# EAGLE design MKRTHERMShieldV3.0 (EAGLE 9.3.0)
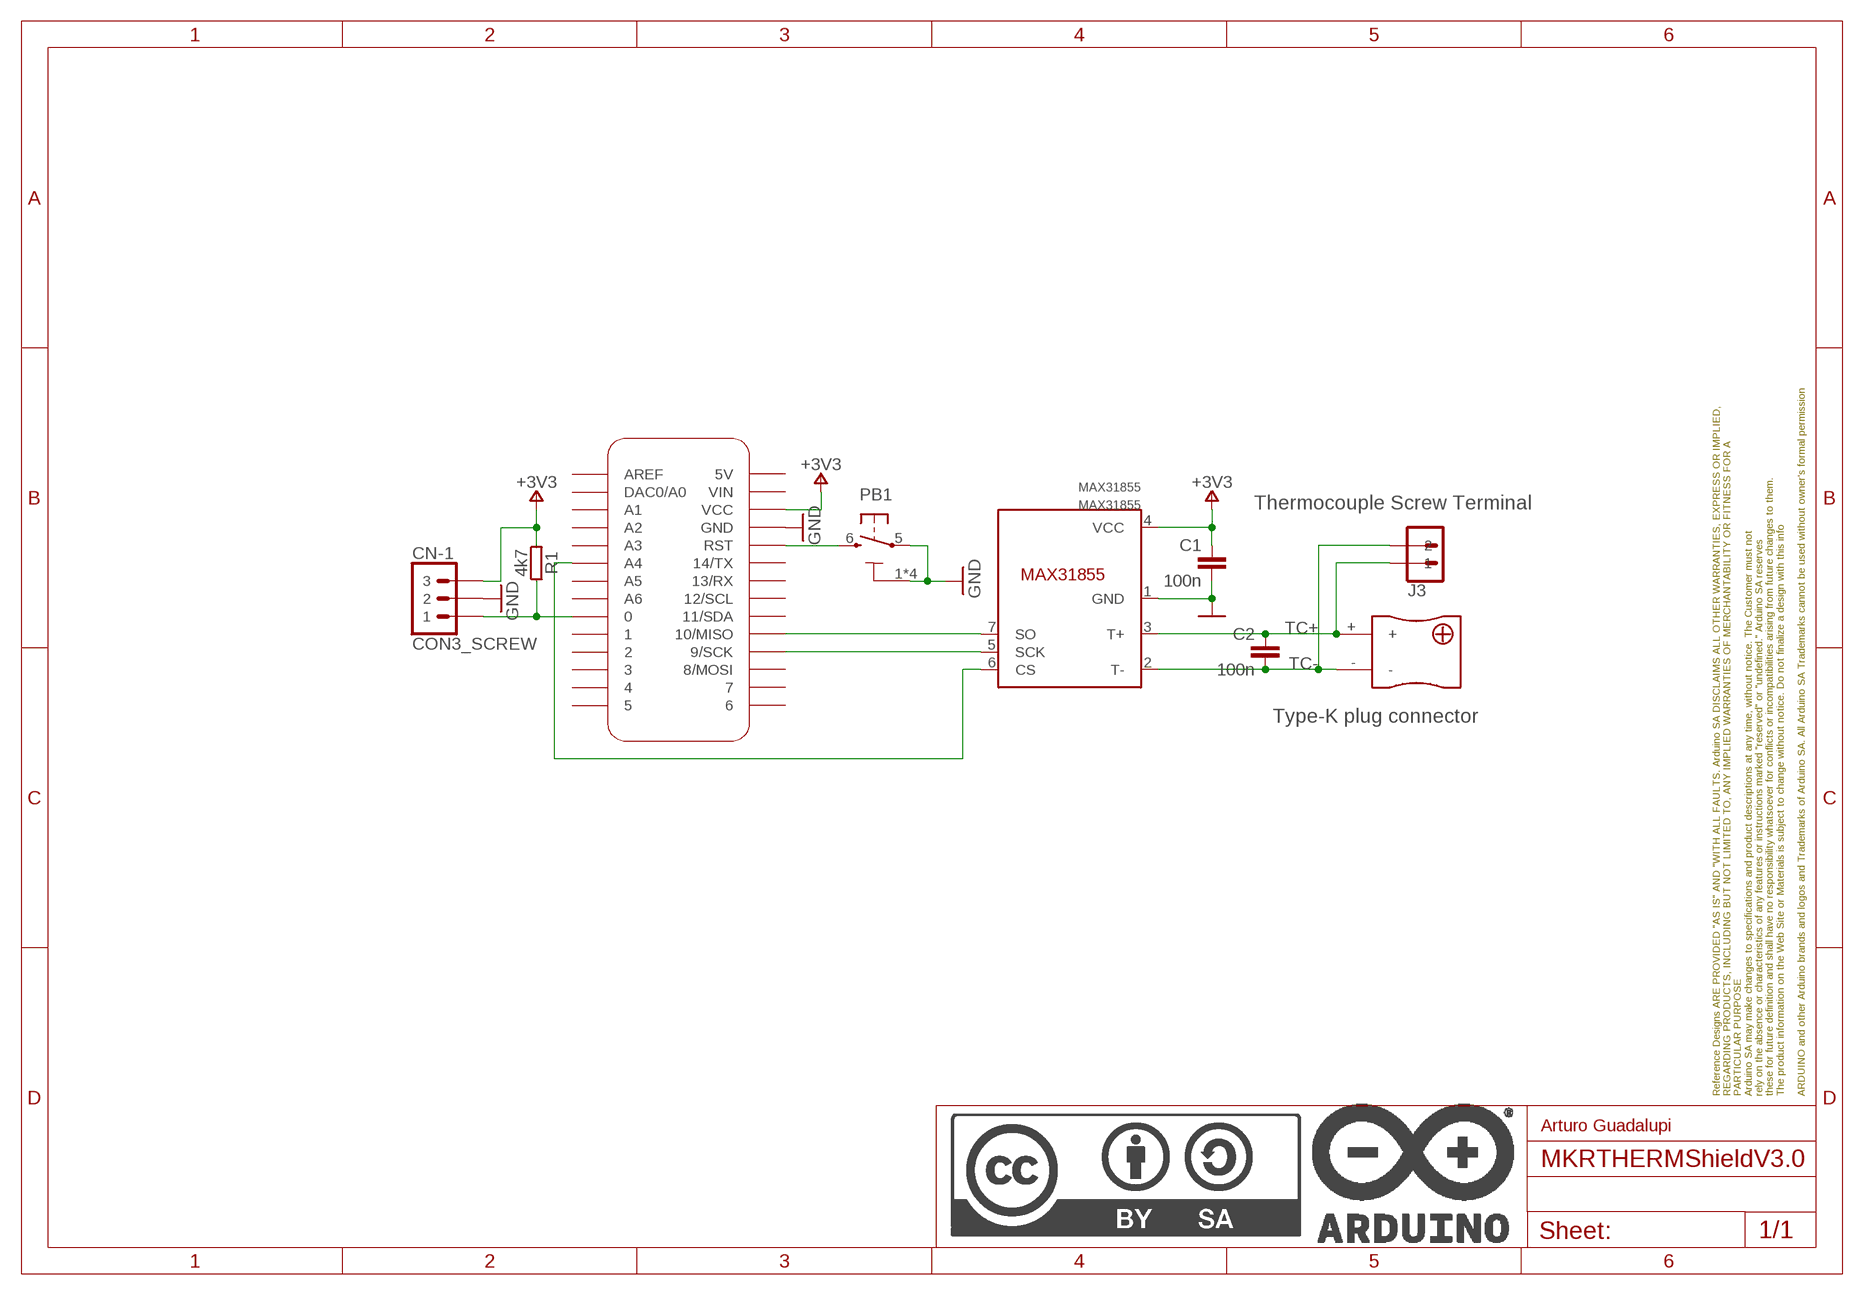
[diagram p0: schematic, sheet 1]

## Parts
C1  100n  C-100NF-0402  [0402-1005X55N]
C2  100n  C-100NF-0402  [0402-1005X55N]
CN-1  CON3_SCREW  SCREW_1X03_254MM  [1X03_2.54_SCREWTERM_FT]
FRAME1  DNP  A4L-LOC  [FRAME]
J3  SCREW2X8.25_  [1X02_8.25_BARRIER-TERMINAL]
MAX31855  MAX31855  [SOIC8]
MKR1  -  MKRBOARD-SHORTTEXT  [MKRBOARD-DIM-SHORTTEXT]
PB1  PTS820  TACTILE1PTS820-NH  [C&K_PTS820_NO_HOLES]
R1  4k7  R-4K7-0402  [0402-1005X55N]
U$1  THERMO_K-PLUG-PCB  [THERMO_K-PLUG-PCB]

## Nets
+3V3: C1.1 CN-1.P$3 MAX31855.4(VCC) MKR1.VCC R1.2
DS18X_DATA: CN-1.P$1 MKR1.0 R1.1
GND: C1.2 CN-1.P$2 MAX31855.1(GND) MKR1.GND PB1.1 PB1.2 PB1.3 PB1.4 PB1.5
MISO: MAX31855.7(SO) MKR1.10(10/MISO)
RESET: MKR1.RST PB1.6
SCK: MAX31855.5(SCK) MKR1.9(9/SCK)
TC+: C2.1 J3.P$1 MAX31855.3(T+) U$1.+
TC-: C2.2 J3.P$2 MAX31855.2(T-) U$1.-
THERMO_CS: MAX31855.6(CS) MKR1.A4
Unconnected: MKR1.1 MKR1.2 MKR1.3 MKR1.4 MKR1.5 MKR1.5V MKR1.6 MKR1.7 MKR1.8(8/MOSI) MKR1.11(11/SDA) MKR1.12(12/SCL) MKR1.13(13/RX) MKR1.14(14/TX) MKR1.A0(DAC0/A0) MKR1.A1 MKR1.A2 MKR1.A3 MKR1.A5 MKR1.A6 MKR1.AREF MKR1.VIN

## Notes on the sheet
- Thermocouple Screw Terminal
- Type-K plug connector
- Arturo Guadalupi

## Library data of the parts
C1 C2 = Arduino-rcl:C: SMD Capacitor; CODE-ARDUINO: 0132; DATASHEET: http://www.tdk.com/pdf/TDKMLCCCapRange.pdf; DISTRIBUTOR-LINK: http://www.digikey.com/product-detail/en/tdk-corporation/C1005X5R1H104K050BB/445-5942-1-ND/2443982; DISTRIBUTOR-PN: 445-5942-1-ND; MANUFACTURER: TDK; MANUFACTURER-PN: C1005X5R1H104K050BB; NOTE: -
CN-1 = Arduino-connectors:SCREW_1X03_254MM; CODE-ARDUINO: -; DATASHEET: http://www.te.com/commerce/DocumentDelivery/DDEController?Action=srchrtrv&DocNm=282834&DocType=Customer+Drawing&DocLang=English; DISTRIBUTOR-LINK: https://www.digikey.com/product-detail/en/te-connectivity-amp-connectors/282834-3/A98334-ND/1153264; DISTRIBUTOR-PN: A98334-ND; MANUFACTURER: TE Connectivity; MANUFACTURER-PN: 282834-3
FRAME1 = Arduino-utility:A4L-LOC; CODE-ARDUINO: DNP; DATASHEET: DNP; DISTRIBUTOR-LINK: DNP; DISTRIBUTOR-PN: DNP; MANUFACTURER: DNP; MANUFACTURER-PN: DNP; NOTE: DNP
J3 = Arduino-connectors:SCREW2X8.25: AdamTech Terminal Barrier 8.25mm pitch; CODE-ARDUINO: A5391; DATASHEET: http://portal.fciconnect.com/Comergent//fci/drawing/yk421xx0x0j0g.pdf; DISTRIBUTOR-LINK: https://www.digikey.com/product-detail/en/amphenol-anytek/YK4210203000G/YK4210203000G-ND/4961594; DISTRIBUTOR-PN: K4210203000G-ND; MANUFACTURER: Amphenol; MANUFACTURER-PN: K4210203000G
MAX31855 = Arduino-Sensors:MAX31855; CODE-ARDUINO: -; DATASHEET: https://datasheets.maximintegrated.com/en/ds/MAX31855.pdf; DISTRIBUTOR-LINK: https://www.digikey.com/product-detail/en/maxim-integrated/MAX31855KASA-T/MAX31855KASA-TCT-ND/2708805; DISTRIBUTOR-PN: MAX31855KASA+TCT-ND; MANUFACTURER: Maxim Integrated; MANUFACTURER-PN: MAX31855KASA+T
MKR1 = Arduino-utility:MKRBOARD: MKR board footprint; CODE-ARDUINO: -; DATASHEET: -; DISTRIBUTOR-LINK: -; DISTRIBUTOR-PN: -; MANUFACTURER: -; MANUFACTURER-PN: -
PB1 = Arduino-pushbuttons:TACTILE1: Tactile Switch SPST-NO Top Actuated Surface Mount; CODE-ARDUINO: 0173; DATASHEET: http://www.ckswitches.com/media/1474/pts820.pdf; DISTRIBUTOR-LINK: https://www.digikey.com/product-detail/en/c-k/PTS820-J15M-SMTR-LFS/CKN10506CT-ND/4176681; DISTRIBUTOR-PN: PTS820 J25K SMTR LFS-ND; MANUFACTURER: C&K; MANUFACTURER-PN: PTS820 J25K SMTR LFS
R1 = Arduino-rcl:R: SMD Resistor; CODE-ARDUINO: 2196; DATASHEET: www.yageo.com.tw/exep/pages/download/literatures/PYu-R_INT-thick_7.pdf; DISTRIBUTOR-LINK: http://www.digikey.com/product-detail/en/yageo/RC0402FR-074K7L/311-4.7KLRCT-ND/2827881; DISTRIBUTOR-PN: 311-4.7KLRCT-ND; MANUFACTURER: Yageo; MANUFACTURER-PN: RC0402FR-074K7L; NOTE: NO
U$1 = Arduino-connectors:THERMO_K-PLUG-PCB; CODE-ARDUINO: A5368; DATASHEET: https://www.labfacility.com/media/attachment/file/pdfs/data-sheet-schematic-im-k-pcb.pdf; DISTRIBUTOR-LINK: http://nl.farnell.com/labfacility/im-k-pcb/socket-mini-pcb-t-c-type-k/dp/3810628?CMP=i-ddd7-00001003; DISTRIBUTOR-PN: 3810628; MANUFACTURER: Lab Facility; MANUFACTURER-PN: IM-K-PCB

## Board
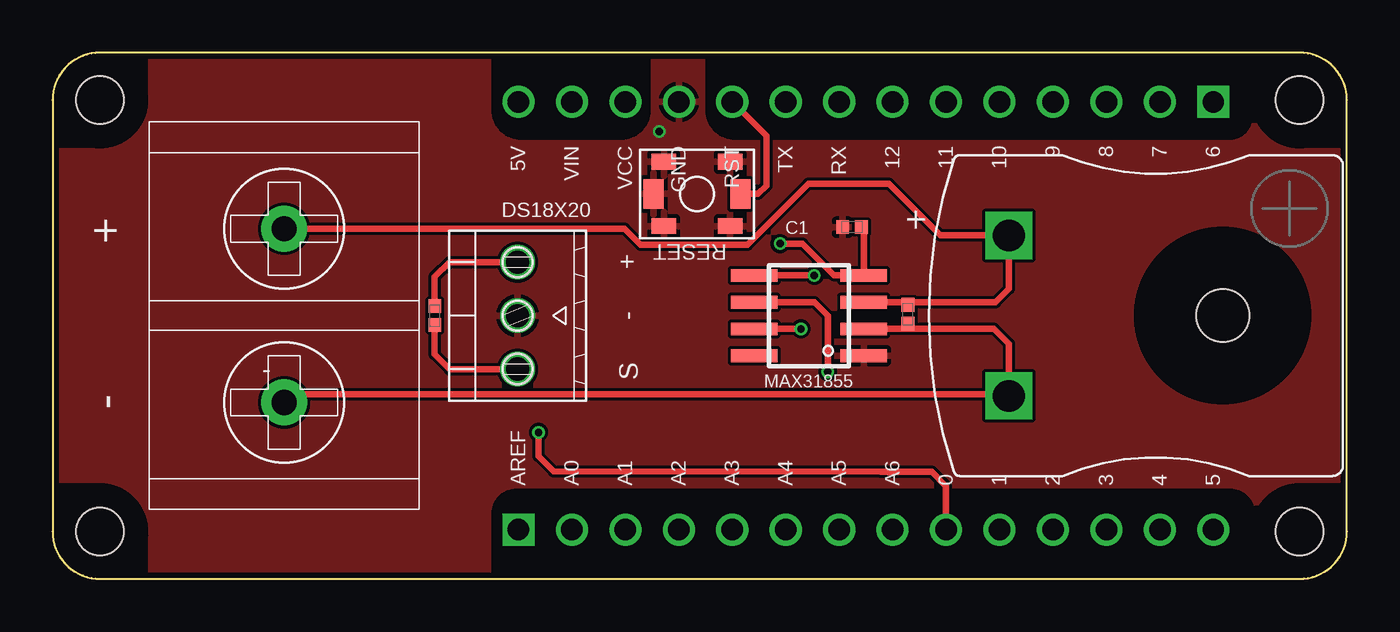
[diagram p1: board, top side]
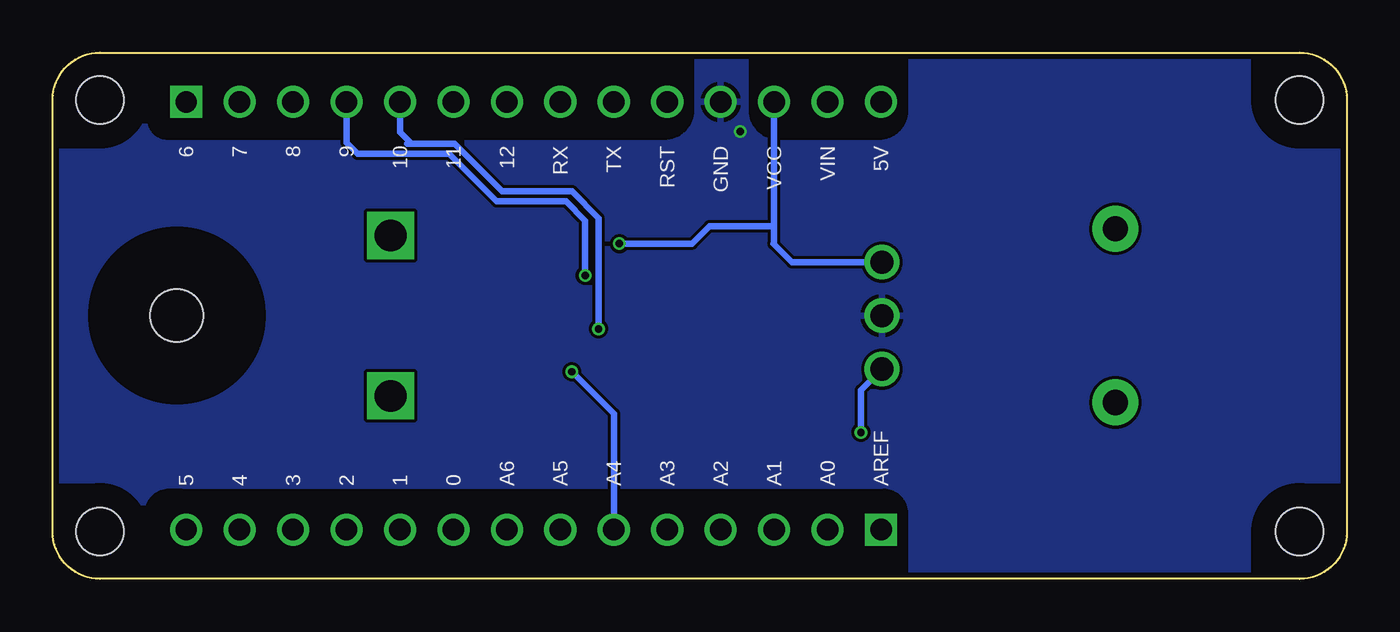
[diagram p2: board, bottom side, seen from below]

Size 61.5 x 25 mm. Coordinates in mm from the lower left corner, seen from the top.
Copper layers (1*16): Top 0.018mm / dielectric 1.55mm / Bottom 0.018mm
Design rules "eC_2Layer_PClass6_BaseCopperO18_eCDefault": minimum track width 0.15mm, minimum drill 0.35mm, track to track 0.15mm, track to pad 0.15mm, pad to pad 0.15mm, via to via 0.15mm, smd to smd 0mil, copper to edge 0.25mm, drill to drill 0.35mm, minimum pad ring 0.175mm, minimum via ring 0.125mm, stop-mask expansion 0mil, vias tented up to drill 0.45mm, thermal gap 0.2mm
tRestrict: area 51.5,8.4 to 59.7,16.6; 15 lines
bRestrict: area 51.5,8.4 to 59.7,16.6; 16 lines

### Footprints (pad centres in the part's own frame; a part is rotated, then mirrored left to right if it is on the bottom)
0402-1005X55N = smd 0.62 x 0.62: 1 -0.45,0; 2 0.45,0
1X03_2.54_SCREWTERM_FT = drill 1.1: P$1 -2.54,0; P$2 0,0; P$3 2.54,0
1X02_8.25_BARRIER-TERMINAL = drill 1.2 pad 2.184: P$1 -4.125,0; P$2 4.125,0
SOIC8 = smd 0.6 x 2.2: 1 -1.905,-2.6; 2 -0.635,-2.6; 3 0.635,-2.6; 4 1.905,-2.6; 5 1.905,2.6; 6 0.635,2.6; 7 -0.635,2.6; 8 -1.905,2.6
MKRBOARD-DIM-SHORTTEXT = drill 1.016 pad 1.524: 0 42.455,2.34; 1 44.995,2.34; 2 47.535,2.34; 3 50.075,2.34; 4 52.615,2.34; 5 55.155,2.34; 5V 22.135,22.66; 7 52.615,22.66; 8 50.075,22.66; 9 47.535,22.66; 10 44.995,22.66; 11 42.455,22.66; 12 39.915,22.66; 13 37.375,22.66; 14 34.835,22.66; A0 24.675,2.34; A1 27.215,2.34; A2 29.755,2.34; A3 32.295,2.34; A4 34.835,2.34; A5 37.375,2.34; A6 39.915,2.34; GND 29.755,22.66; RST 32.295,22.66; VCC 27.215,22.66; VIN 24.675,22.66 | drill 1.016 pad 1.524 square: 6 55.155,22.66; AREF 22.135,2.34 | hole 2.25: 59.25,2.25; 59.25,22.75; 2.25,2.25; 2.25,22.75
C&K_PTS820_NO_HOLES = smd 1.15 x 0.75: 1 -1.575,1.525; 2 -1.575,-1.525; 3 1.575,1.525; 4 1.575,-1.525 | smd 0.95 x 1.4: 5 -2.075,0; 6 2.075,0
THERMO_K-PLUG-PCB = drill 1.5 square: + -3.81,0; - 3.81,0 | hole 2.5: 0,10.16

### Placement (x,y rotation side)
C1  37.99,16.71 180 top
C2  40.64,12.57 270 top
CN-1  22.09,12.51 90 top
FRAME1  0,0 0 top
J3  11,12.51 270 top
MAX31855  35.94,12.51 90 top
MKR1  0,0 0 top
PB1  30.62,18.29 0 top
R1  18.16,12.51 90 top
U$1  45.44,12.51 270 top

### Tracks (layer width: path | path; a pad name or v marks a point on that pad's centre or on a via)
+3V3  (via drill 0.35)
  Top 0.305: v34.57,15.93 35.64,15.93 37.13,14.43 38.55,14.43 MAX31855.4 38.54,16.71 C1.1 | CN-1.P$3 18.86,15.05 18.16,14.35 R1.2
  Bottom 0.305: 27.21,19.77 MKR1.VCC 27.21,16.76 | 27.21,16.76 27.21,15.95 27.24,15.93 26.36,15.05 CN-1.P$3 | v34.57,15.93 31.13,15.93 30.29,16.76 27.21,16.76
DS18X_DATA  (via drill 0.35)
  Top 0.305: 39.37,5.08 23.8,5.11 23.09,5.82 v23.09,6.96 | 39.37,5.08 39.72,5.08 | CN-1.P$1 18.86,9.97 18.16,10.67 R1.1 | 39.37,5.08 41.78,5.08 42.45,4.41 MKR1.0
  Bottom 0.305: v23.09,6.96 23.09,8.97 CN-1.P$1
GND  (via drill 0.35)
  other vias: 28.83,21.26
  pour Top: 2.54,25.02 59.18,25.02 arc-90 61.72,22.48 61.72,2.54 arc-90 59.18,0 2.54,0 arc-90 0,2.54 0,22.48 arc-90
  pour Bottom: 2.54,25.02 59.18,25.02 arc-90 61.72,22.48 61.72,2.54 arc-90 59.18,0 2.54,0 arc-90 0,2.54 0,22.48 arc-90
MISO  (via drill 0.35)
  Top 0.305: MAX31855.7 v35.56,11.87
  Bottom 0.305: 44.45,20.67 42.4,20.67 40.14,18.41 36.83,18.41 35.56,17.14 v35.56,11.87 | 44.45,20.67 44.65,20.67 | 44.45,20.67 44.99,21.22 MKR1.10
RESET
  Top 0.305: PB1.6 33.53,18.29 33.91,18.67 33.91,21.05 MKR1.RST
SCK  (via drill 0.35)
  Top 0.305: MAX31855.5 v36.2,14.41
  Bottom 0.305: MKR1.9 47.53,20.71 47.02,20.19 42.67,20.19 40.41,17.93 37.11,17.93 36.2,17.02 v36.2,14.41
TC+
  Top 0.305: MAX31855.3 40.64,13.14 | 40.64,13.14 44.81,13.14 45.44,13.78 U$1.+ 42.2,16.32 39.73,18.78 35.92,18.78 33.02,15.88 27.94,15.88 27.18,16.63 J3.P$1 | C2.1 40.64,13.14
TC-
  Top 0.152: J3.P$2 11,8.76
  Top 0.305: MAX31855.2 40.64,11.87 | 40.64,11.87 44.73,11.87 45.44,11.16 U$1.- 45.38,8.76 11,8.76 | C2.2 40.64,11.87
THERMO_CS  (via drill 0.35)
  Top 0.305: MAX31855.6 36.2,13.14 36.83,12.51 v36.83,9.84
  Bottom 0.305: MKR1.A4 34.84,7.85 v36.83,9.84

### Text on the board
tPlace: + | DS18X20 | RESET | + | - | - | S | -

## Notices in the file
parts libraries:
Arduino-utility: Copyright (c) 2016-2017 Arduino LLC. All right reserved.
